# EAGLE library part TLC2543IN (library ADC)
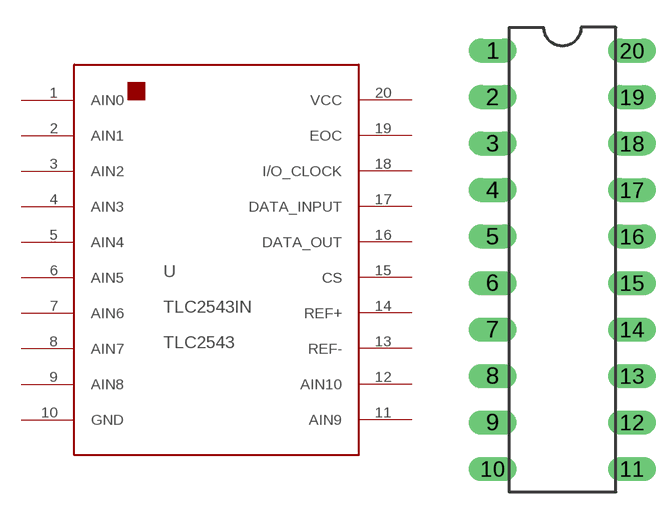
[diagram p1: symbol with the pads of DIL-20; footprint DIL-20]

Designator prefix -

## TLC2543IN  [DIL-20]
1  AIN0
2  AIN1
3  AIN2
4  AIN3
5  AIN4
6  AIN5
7  AIN6
8  AIN7
9  AIN8
10  GND
11  AIN9
12  AIN10
13  REF-
14  REF+
15  CS
16  DATA_OUT
17  DATA_INPUT
18  I/O_CLOCK
19  EOC
20  VCC

## Footprint DIL-20 (pad centres in mm)
drill 0.813 long: 1 -8.89,6.35; 2 -8.89,3.81; 3 -8.89,1.27; 4 -8.89,-1.27; 5 -8.89,-3.81; 6 -8.89,-6.35; 7 -8.89,-8.89; 8 -8.89,-11.43; 9 -8.89,-13.97; 10 -8.89,-16.51; 11 -1.27,-16.51; 12 -1.27,-13.97; 13 -1.27,-11.43; 14 -1.27,-8.89; 15 -1.27,-6.35; 16 -1.27,-3.81; 17 -1.27,-1.27; 18 -1.27,1.27; 19 -1.27,3.81; 20 -1.27,6.35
